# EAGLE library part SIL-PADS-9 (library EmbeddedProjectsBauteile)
Anschlüsse 2,54mm Raster, SMT oder THT
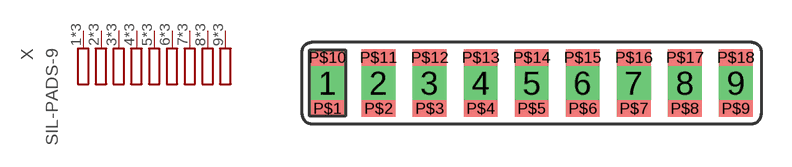
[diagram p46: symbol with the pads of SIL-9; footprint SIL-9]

Designator prefix X

## SIL-PADS-9  [SIL-9]
1  1  pas
2  2  pas
3  3  pas
4  4  pas
5  5  pas
6  6  pas
7  7  pas
8  8  pas
9  9  pas
P$1  1  pas
P$2  2  pas
P$3  3  pas
P$4  4  pas
P$5  5  pas
P$6  6  pas
P$7  7  pas
P$8  8  pas
P$9  9  pas
P$10  1  pas
P$11  2  pas
P$12  3  pas
P$13  4  pas
P$14  5  pas
P$15  6  pas
P$16  7  pas
P$17  8  pas
P$18  9  pas

## Footprint SIL-9 (pad centres in mm)
drill 0.813 pad 1.676 square: 1 0,0; 2 2.54,0; 3 5.08,0; 4 7.62,0; 5 10.16,0; 6 12.7,0; 7 15.24,0; 8 17.78,0; 9 20.32,0
smd 1.676 x 0.813: P$1 0,-1.27; P$2 2.54,-1.27; P$3 5.08,-1.27; P$4 7.62,-1.27; P$5 10.16,-1.27; P$6 12.7,-1.27; P$7 15.24,-1.27; P$8 17.78,-1.27; P$9 20.32,-1.27; P$10 0,1.27; P$11 2.54,1.27; P$12 5.08,1.27; P$13 7.62,1.27; P$14 10.16,1.27; P$15 12.7,1.27; P$16 15.24,1.27; P$17 17.78,1.27; P$18 20.32,1.27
